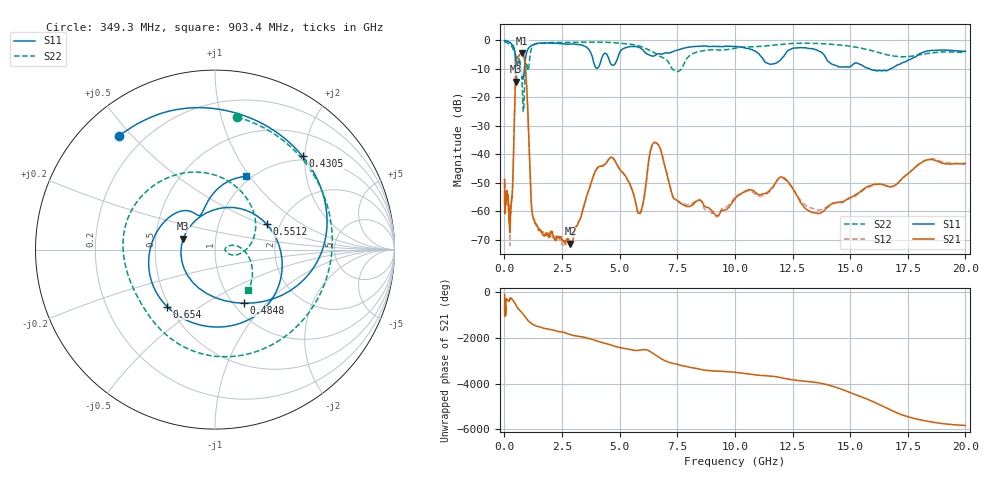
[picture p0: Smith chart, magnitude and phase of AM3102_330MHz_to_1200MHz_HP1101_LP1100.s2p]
! Date/Time: Tue, Sep 11, 2018 5:22 PM
! Network Analyzer: Agilent Technologies E8362B Rev: A.07.50.63
! Sweep from 0.010 to 20.000 GHz, 1601 Points, Sweep Type: LOG
! Power Supply: 4.949 V, 0.001 A
# Hz S DB R 50
!freq MagS11 AngS11 MagS21 AngS21 MagS12 AngS12 MagS22 AngS22
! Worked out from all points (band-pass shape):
!   1601 points, 10 MHz to 20 GHz, reference 50 ohm
!   highest |S21| = -4.45 dB at 765 MHz (marker M1); lowest = -71.4 dB at 2.866 GHz (marker M2)
!   |S21| within 3 dB of the highest: 516.3 MHz to 884.1 MHz (367.8 MHz wide, 52.5 % of centre)
!   lowest |S11| = -14.6 dB at 513.3 MHz (marker M3), VSWR 1.46, Z = 34.7 + j4.38 ohm
!   |S11| at or under -10 dB: 486.9 MHz to 550 MHz (63.1 MHz wide, 12.2 % of centre); 728.8 MHz to 867.8 MHz (139 MHz wide, 17.4 % of centre); 15.86 GHz to 16.75 GHz (892 MHz wide, 5.47 % of centre)
!   |S22| runs from -25.0 to -0.2 dB; largest |S21 - S12| = 0.0094
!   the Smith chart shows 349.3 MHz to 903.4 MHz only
!   S11 on the Smith chart (normalised r, x): 349.3 MHz: 0.11, +0.46; 430.5 MHz: 0.92, +1.95; 484.8 MHz: 1.12, -0.76; 551.2 MHz: 1.70, +0.54; 654 MHz: 0.49, -0.37; 903.4 MHz: 0.94, +0.96
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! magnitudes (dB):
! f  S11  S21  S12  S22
! 10 MHz  0.0  -49.0  -57.6  -0.2
! 35.55 MHz  -0.1  -58.6  -60.0  -0.5
! 126.4 MHz  -0.2  -54.1  -54.4  -0.9
! 237.7 MHz  -0.7  -67.0  -72.1  -1.4
! 349.3 MHz  -1.6  -53.1  -53.7  -2.5
! 430.5 MHz  -2.9  -27.2  -27.2  -4.0
! 447.2 MHz  -3.6  -21.8  -21.8  -4.1
! 484.8 MHz  -9.4  -11.7  -11.7  -5.0
! 513.3 MHz  -14.6  -7.7  -7.8  -5.8
! 551.2 MHz  -9.9  -6.3  -6.3  -5.9
! 654 MHz  -7.6  -5.1  -5.2  -6.8
! 765 MHz  -11.6  -4.5  -4.5  -14.2
! 825.4 MHz  -13.4  -5.0  -5.1  -25.0
! 903.4 MHz  -7.1  -8.9  -9.0  -10.6
! 1.196 GHz  -1.7  -60.1  -60.0  -2.4
! 1.59 GHz  -1.0  -67.3  -67.2  -0.9
! 2.866 GHz  -1.2  -71.4  -69.8  -0.7
! 4.564 GHz  -7.3  -41.5  -41.3  -0.7
! 5.652 GHz  -2.1  -55.4  -55.6  -1.6
! 6.549 GHz  -5.2  -35.8  -36.0  -4.6
! 9.004 GHz  -2.1  -59.9  -60.8  -3.3
! 20 GHz  -3.8  -43.2  -43.6  -4.2
